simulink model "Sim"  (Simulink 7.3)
settings: Solver=ode45  StartTime=0.0  StopTime=22  RelTol=1e-3
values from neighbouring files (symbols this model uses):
  d2r = pi/180    (= 0.0174532925199)    [run.m]    (also in LQR_Des.m)
  r2d = 1/d2r    (= 57.2957795131)    [run.m]    (also in LQR_Des.m)
undefined symbols (not defined in the file or in its folder): Av, Bv, Cv, Dv, Kmix, Kpr, Kq

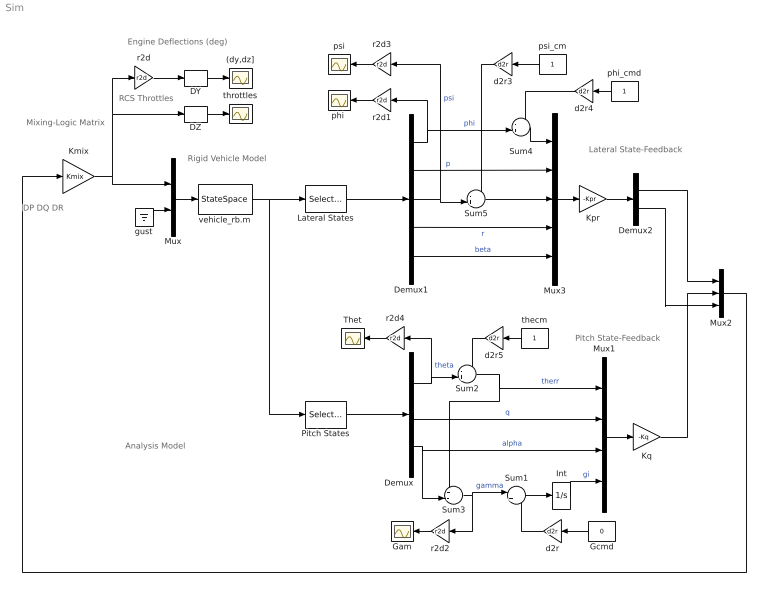
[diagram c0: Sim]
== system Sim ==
  note: Analysis Model
  note: Rigid Vehicle Model
  note: Pitch State-Feedback
  note: Lateral State-Feedback
  note: Mixing-Logic Matrix
  note: Engine Deflections (deg)
  note: RCS Throttles
  note: DP DQ DR
  (dy,dz] : Scope
  DY : Selector  InputPortWidth=4  IndexOptions=Index vector (dialog)  Indices=[1,2]  OutputSizes=1
  DZ : Selector  InputPortWidth=4  IndexOptions=Index vector (dialog)  Indices=[1,2]  OutputSizes=1
  Demux : Demux  Outputs=3
  Demux1 : Demux  Outputs=5
  Demux2 : Demux  Outputs=2
  Gam : Scope
  Gcmd : Constant  Value=0  OutDataType=fixdt(1, 16)  OutScaling=2^0
  Int : Integrator
  Kmix : Gain  Gain=Kmix  Multiplication=Matrix(K*u)  ParameterDataType=fixdt(1, 16)  ParameterScaling=2^0  OutDataType=fixdt(1, 16)  OutScaling=2^0
  Kpr : Gain  Gain=-Kpr  Multiplication=Matrix(K*u)  ParameterDataType=fixdt(1, 16)  ParameterScaling=2^0  OutDataType=fixdt(1, 16)  OutScaling=2^0
  Kq : Gain  Gain=-Kq  Multiplication=Matrix(K*u)  ParameterDataType=fixdt(1, 16)  ParameterScaling=2^0  OutDataType=fixdt(1, 16)  OutScaling=2^0
  Lateral States : Selector  InputPortWidth=14  IndexOptions=Index vector (dialog)  Indices=[1,2, 5,6, 8]  OutputSizes=1
  Mux : Mux  Inputs=[4,1]
  Mux1 : Mux
  Mux2 : Mux  Inputs=3
  Mux3 : Mux  Inputs=5
  Pitch States : Selector  InputPortWidth=14  IndexOptions=Index vector (dialog)  Indices=[3, 4, 7]  OutputSizes=1
  Sum1 : Sum  Inputs=|+-  OutDataType=sfix(16)  OutScaling=2^0
  Sum2 : Sum  Inputs=-+|  OutDataType=sfix(16)  OutScaling=2^0
  Sum3 : Sum  Inputs=+-|  OutDataType=sfix(16)  OutScaling=2^0
  Sum4 : Sum  Inputs=-+|  OutDataType=sfix(16)  OutScaling=2^0
  Sum5 : Sum  Inputs=-+|  OutDataType=sfix(16)  OutScaling=2^0
  Thet : Scope
  d2r{,3..5} (4 alike) : Gain  Gain=d2r  ParameterDataType=fixdt(1, 16)  ParameterScaling=2^0  OutDataType=fixdt(1, 16)  OutScaling=2^0
  gust : Ground
  "phi " : Scope
  phi_cmd : Constant  OutDataType=fixdt(1, 16)  OutScaling=2^0
  psi : Scope
  psi_cm : Constant  OutDataType=fixdt(1, 16)  OutScaling=2^0
  r2d{,1..4} (5 alike) : Gain  Gain=r2d  ParameterDataType=fixdt(1, 16)  ParameterScaling=2^0  OutDataType=fixdt(1, 16)  OutScaling=2^0
  thecm : Constant  OutDataType=fixdt(1, 16)  OutScaling=2^0
  throttles : Scope
  vehicle_rb.m : StateSpace  A=Av  B=Bv  C=Cv  D=Dv
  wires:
  Mux/1 -> vehicle_rb.m/1
  Kmix/1 -> Mux/1, DZ/1, r2d/1
  gust/1 -> Mux/2
  vehicle_rb.m/1 -> Pitch States/1, Lateral States/1
  Demux/2 -> Mux1/2  "q"
  Demux/3 -> Mux1/3, Sum3/2  "alpha"
  Pitch States/1 -> Demux/1
  Mux1/1 -> Kq/1
  Demux/1 -> Sum2/2, r2d4/1  "theta"
  Sum2/1 -> Mux1/1, Sum3/1  "therr"
  thecm/1 -> d2r5/1
  Kq/1 -> Mux2/2
  Int/1 -> Mux1/4  "gi"
  Gcmd/1 -> d2r/1
  Sum1/1 -> Int/1
  Sum3/1 -> Sum1/1, r2d2/1  "gamma"
  Demux1/2 -> Mux3/2  "p"
  Lateral States/1 -> Demux1/1
  Mux3/1 -> Kpr/1
  Demux1/4 -> Mux3/4  "r"
  psi_cm/1 -> d2r3/1
  Demux1/5 -> Mux3/5  "beta"
  Demux1/3 -> Sum5/2, r2d3/1  "psi"
  Sum5/1 -> Mux3/3
  Kpr/1 -> Demux2/1
  Demux2/1 -> Mux2/1
  Demux2/2 -> Mux2/3
  Sum4/1 -> Mux3/1
  Demux1/1 -> Sum4/2, r2d1/1  "phi"
  phi_cmd/1 -> d2r4/1
  Mux2/1 -> Kmix/1
  DZ/1 -> throttles/1
  DY/1 -> (dy,dz]/1
  d2r3/1 -> Sum5/1
  d2r4/1 -> Sum4/1
  d2r/1 -> Sum1/2
  d2r5/1 -> Sum2/1
  r2d3/1 -> psi/1
  r2d1/1 -> "phi "/1
  r2d2/1 -> Gam/1
  r2d4/1 -> Thet/1
  r2d/1 -> DY/1
